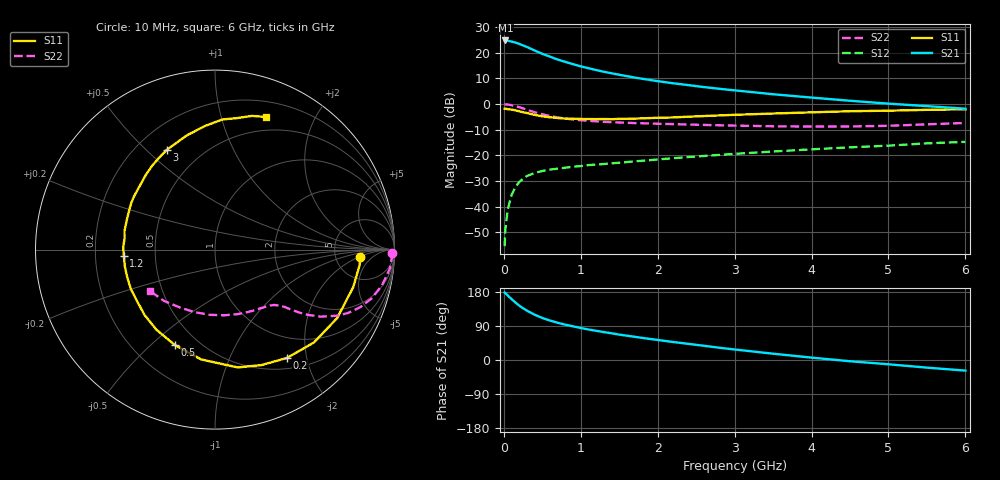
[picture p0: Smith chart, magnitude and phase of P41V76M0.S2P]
! SIEMENS Small Signal Semiconductors
! BFP182
! Si NPN RF Bipolar Junction Transistor in SOT143
! VCE = 1.75 V  IC = 6 mA
! Common Emitter S-Parameters:  March  1996
# GHz  S  MA  R  50
!  f  S11  S21  S12  S22
! GHz  MAG  ANG  MAG  ANG  MAG  ANG  MAG  ANG
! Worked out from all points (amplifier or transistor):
!   36 points, 10 MHz to 6 GHz, reference 50 ohm
!   highest |S21| = 24.8 dB at 20 MHz (marker M1)
!   |S21| within 3 dB of that: start of sweep to 333.7 MHz
!   unconditionally stable (mu >= 1): 1.409 GHz to 5.476 GHz
!   at 250 MHz: K = 0.24, MSG = 26.0 dB, |S12| = -29.1 dB
!   at 1.4 GHz: K = 1.00, MSG = 17.5 dB, |S12| = -23.1 dB
!   at 6 GHz: K = 0.95, MSG = 6.5 dB, |S12| = -14.7 dB
!   S11 on the Smith chart (normalised r, x): 10 MHz: 8.94, -2.20; 200 MHz: 0.66, -1.67; 500 MHz: 0.37, -0.60; 1.2 GHz: 0.33, -0.03; 3 GHz: 0.32, +0.58; 6 GHz: 0.35, +1.39
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0.01  0.8093 -3.0  17.28 178.2  0.0017 82.4  0.9878 -1.2
0.02  0.8106 -6.0  17.39 176.5  0.0036 83.4  0.9863 -2.5
0.05  0.7981 -15.2  17.21 170.2  0.0087 82.5  0.9803 -6.2
0.1  0.7802 -29.3  16.54 160.8  0.0169 74.3  0.9516 -12.1
0.15  0.7561 -43.2  15.81 151.9  0.024 67.7  0.9132 -17.4
0.2  0.7249 -56.3  14.92 143.6  0.0302 63.1  0.8696 -21.7
0.25  0.6938 -68.0  13.88 136.4  0.035 57.7  0.8221 -25.4
0.3  0.6686 -79.1  12.97 130.4  0.0396 53.7  0.7745 -28.4
0.4  0.6168 -97.2  11.09 119.5  0.0455 47.4  0.6951 -32.5
0.5  0.5764 -112.9  9.541 111.0  0.0496 42.8  0.6327 -35.1
0.6  0.5532 -126.0  8.407 104.1  0.0529 40.7  0.5856 -36.8
0.7  0.5358 -137.0  7.377 98.3  0.0552 38.4  0.5488 -37.9
0.9  0.5178 -154.7  5.99 88.8  0.0602 36.7  0.5014 -39.5
1.1  0.5109 -169.3  5.007 80.5  0.0646 35.8  0.4719 -41.3
1.2  0.5095 -176.2  4.606 77.1  0.0662 35.5  0.4613 -42.2
1.7  0.5209 158.9  3.293 61.3  0.0764 35.8  0.4264 -47.8
2.2  0.5492 139.8  2.545 47.5  0.088 35.2  0.4073 -55.3
3  0.6173 115.8  1.852 27.8  0.1071 32.8  0.3807 -70.9
3.5  0.6545 104.1  1.555 16.6  0.119 30.2  0.3693 -82.3
4.5  0.726 86.8  1.161 -3.3  0.1435 24.7  0.3665 -108.3
5.5  0.7726 74.6  0.912 -20.1  0.1718 18.6  0.403 -134.8
6  0.7912 69.1  0.813 -28.0  0.1835 14.0  0.4289 -147.4
